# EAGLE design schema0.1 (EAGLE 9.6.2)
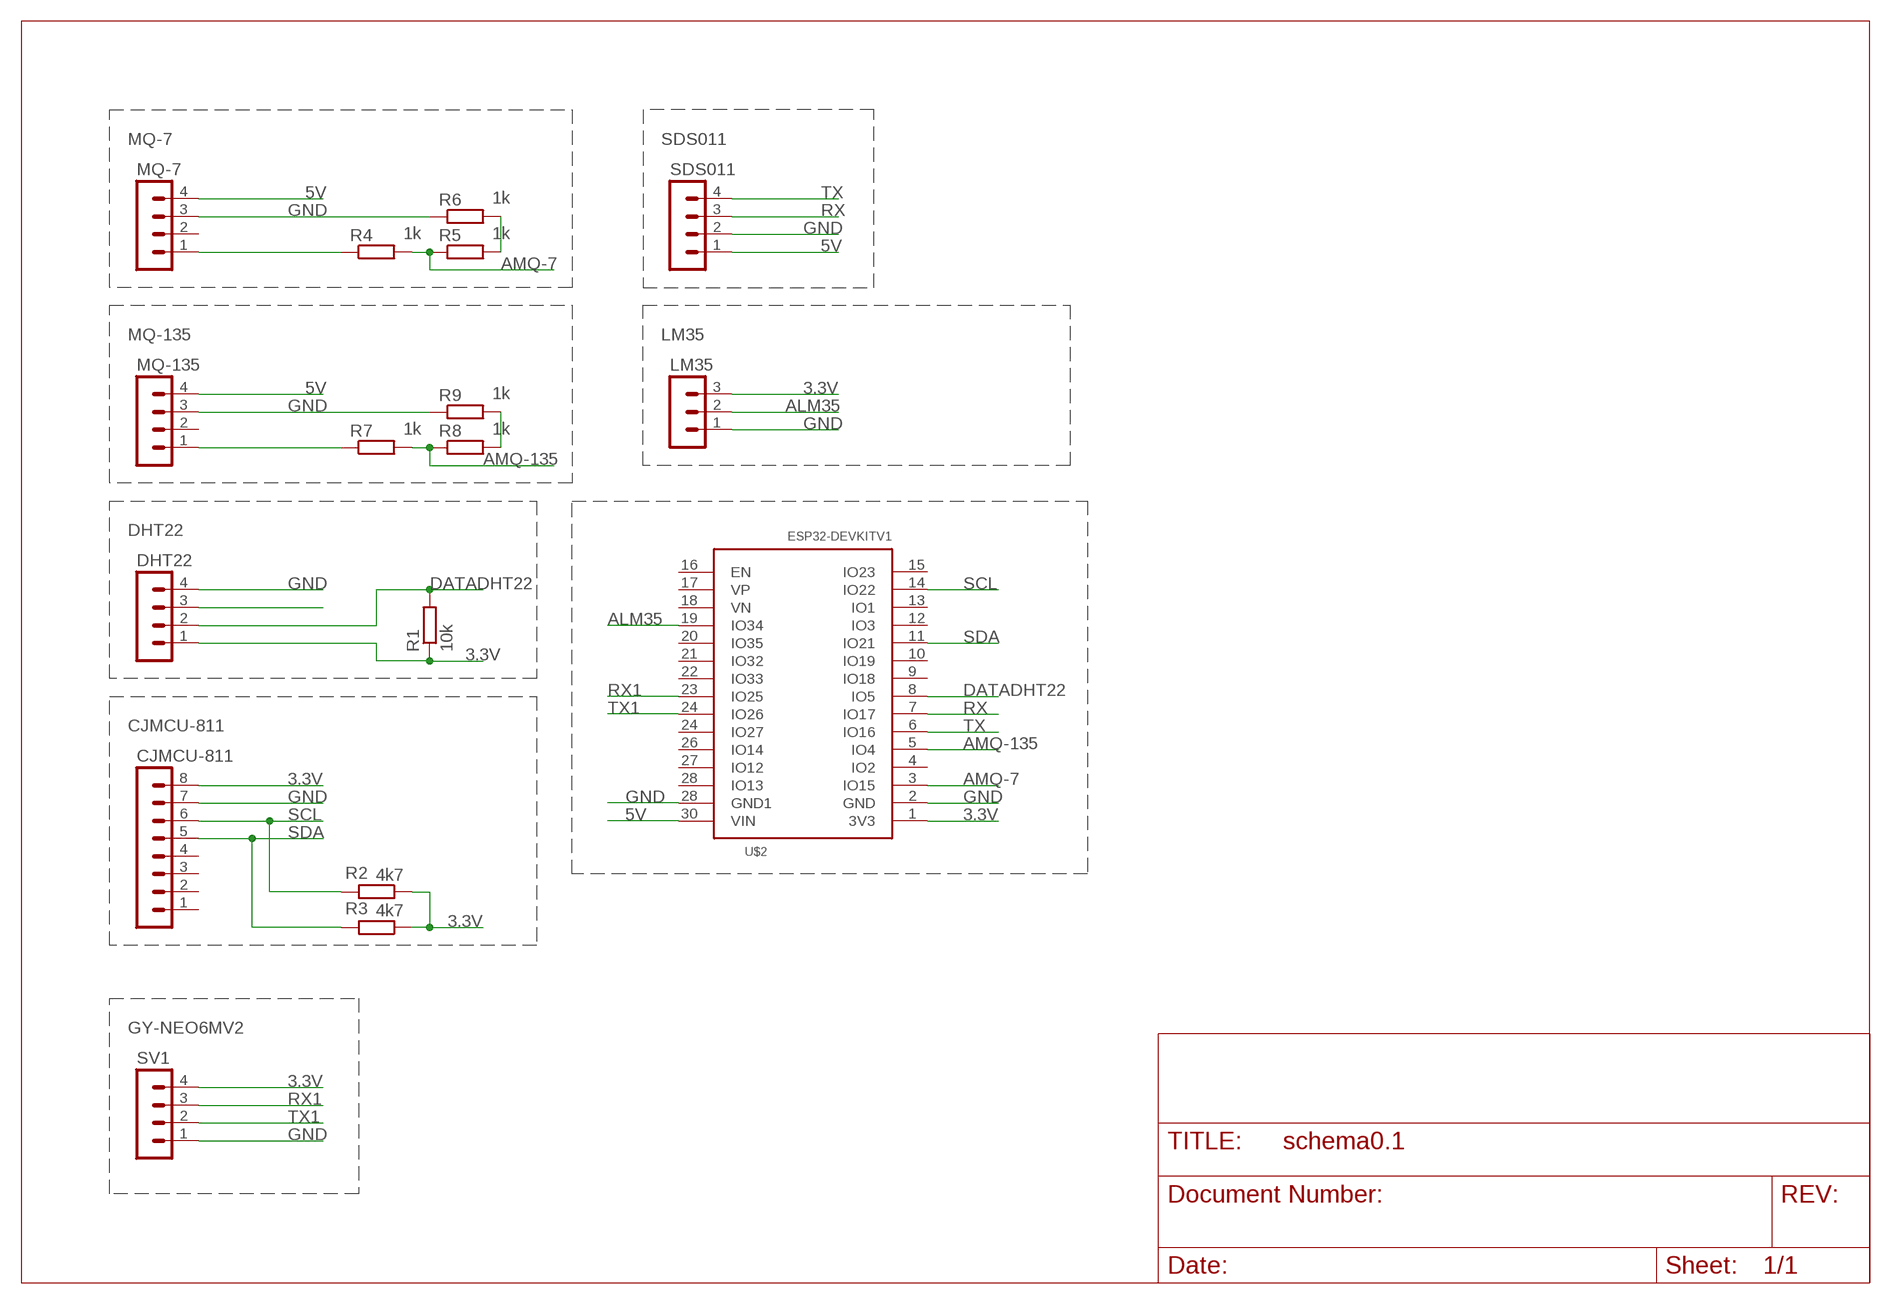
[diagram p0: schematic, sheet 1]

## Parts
CJMCU-811  MA08-1  [MA08-1]
DHT22  MA04-1  [MA04-1]
LM35  MA03-1  [MA03-1]
MQ-7  MA04-1  [MA04-1]
MQ-135  MA04-1  [MA04-1]
R1  10k  R-EU_0207/10  [0207/10]
R2  4k7  R-EU_0207/10  [0207/10]
R3  4k7  R-EU_0207/10  [0207/10]
R4  1k  R-EU_0207/10  [0207/10]
R5  1k  R-EU_0207/10  [0207/10]
R6  1k  R-EU_0207/10  [0207/10]
R7  1k  R-EU_0207/10  [0207/10]
R8  1k  R-EU_0207/10  [0207/10]
R9  1k  R-EU_0207/10  [0207/10]
SDS011  MA04-1  [MA04-1]
SV1  MA04-1  [MA04-1]
U$2  ESP32DEVKITV1  [ESP32-DEVKITV1]

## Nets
0: MQ-7.1 R4.1
1: MQ-135.1 R7.1
3.3V: CJMCU-811.8 DHT22.1 LM35.3 R1.1 R2.1 R3.1 SV1.4 U$2.1(3V3)
5V: MQ-7.4 MQ-135.4 SDS011.1 U$2.30(VIN)
ALM35: LM35.2 U$2.19(IO34)
AMQ-7: R4.2 R5.1 U$2.3(IO15)
AMQ-135: R7.2 R8.1 U$2.5(IO4)
DATADHT22: DHT22.2 R1.2 U$2.8(IO5)
GND: CJMCU-811.7 DHT22.4 LM35.1 MQ-7.3 MQ-135.3 R6.1 R9.1 SDS011.2 SV1.1 U$2.2(GND) U$2.28(GND1)
N$1: R8.2 R9.2
N$2: R5.2 R6.2
N$14: DHT22.3
RX: SDS011.3 U$2.7(IO17)
RX1: SV1.3 U$2.23(IO25)
SCL: CJMCU-811.6 R2.2 U$2.14(IO22)
SDA: CJMCU-811.5 R3.2 U$2.11(IO21)
TX: SDS011.4 U$2.6(IO16)
TX1: SV1.2 U$2.24(IO26)
Unconnected: CJMCU-811.1 CJMCU-811.2 CJMCU-811.3 CJMCU-811.4 MQ-7.2 MQ-135.2 U$2.4(IO2) U$2.9(IO18) U$2.10(IO19) U$2.12(IO3) U$2.13(IO1) U$2.15(IO23) U$2.16(EN) U$2.17(VP) U$2.18(VN) U$2.20(IO35) U$2.21(IO32) U$2.22(IO33) U$2.24(IO27) U$2.26(IO14) U$2.27(IO12) U$2.28(IO13)

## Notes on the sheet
- MQ-7 | SDS011
- MQ-135 | LM35
- DHT22
- CJMCU-811
- GY-NEO6MV2

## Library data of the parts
CJMCU-811 = con-lstb:MA08-1: PIN HEADER; OC_FARNELL: unknown; OC_NEWARK: unknown
DHT22 MQ-7 MQ-135 SDS011 SV1 = con-lstb:MA04-1: PIN HEADER; OC_FARNELL: unknown; OC_NEWARK: unknown
LM35 = con-lstb:MA03-1: PIN HEADER; OC_FARNELL: unknown; OC_NEWARK: unknown
R1-R9 = rcl:R-EU_: RESISTOR, European symbol; SPICEPREFIX: R
U$2 = ESP32-DEVKITV1:ESP32DEVKITV1

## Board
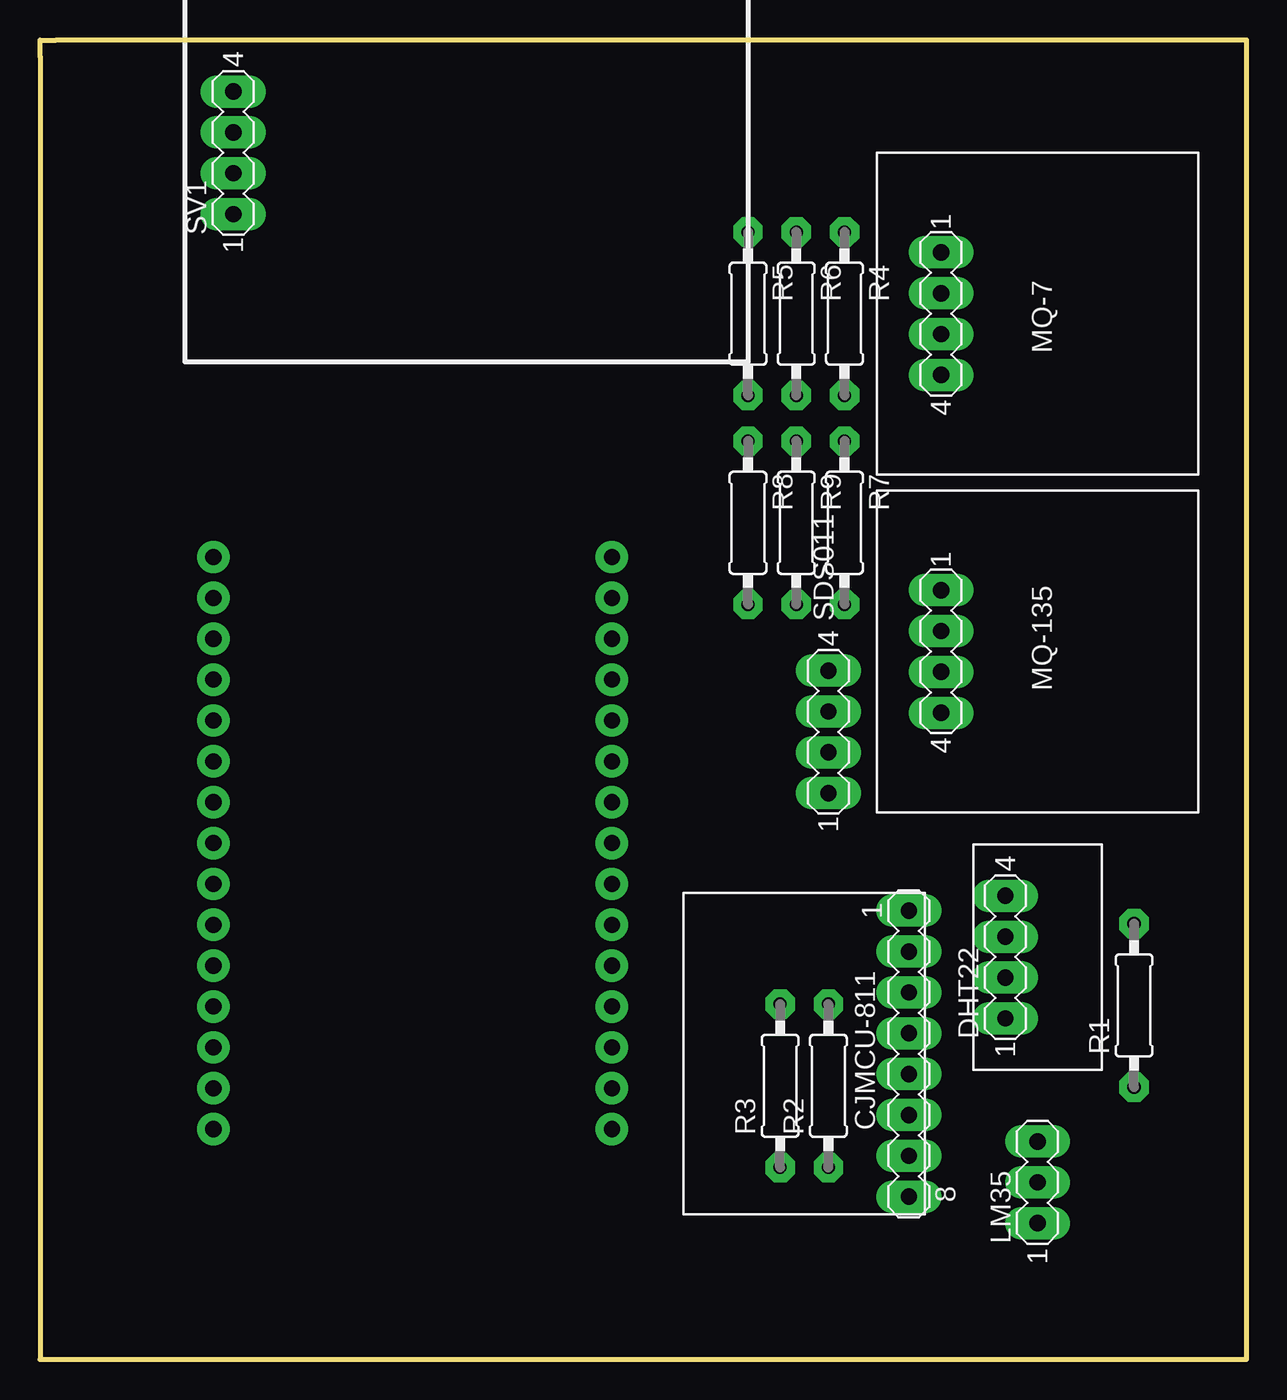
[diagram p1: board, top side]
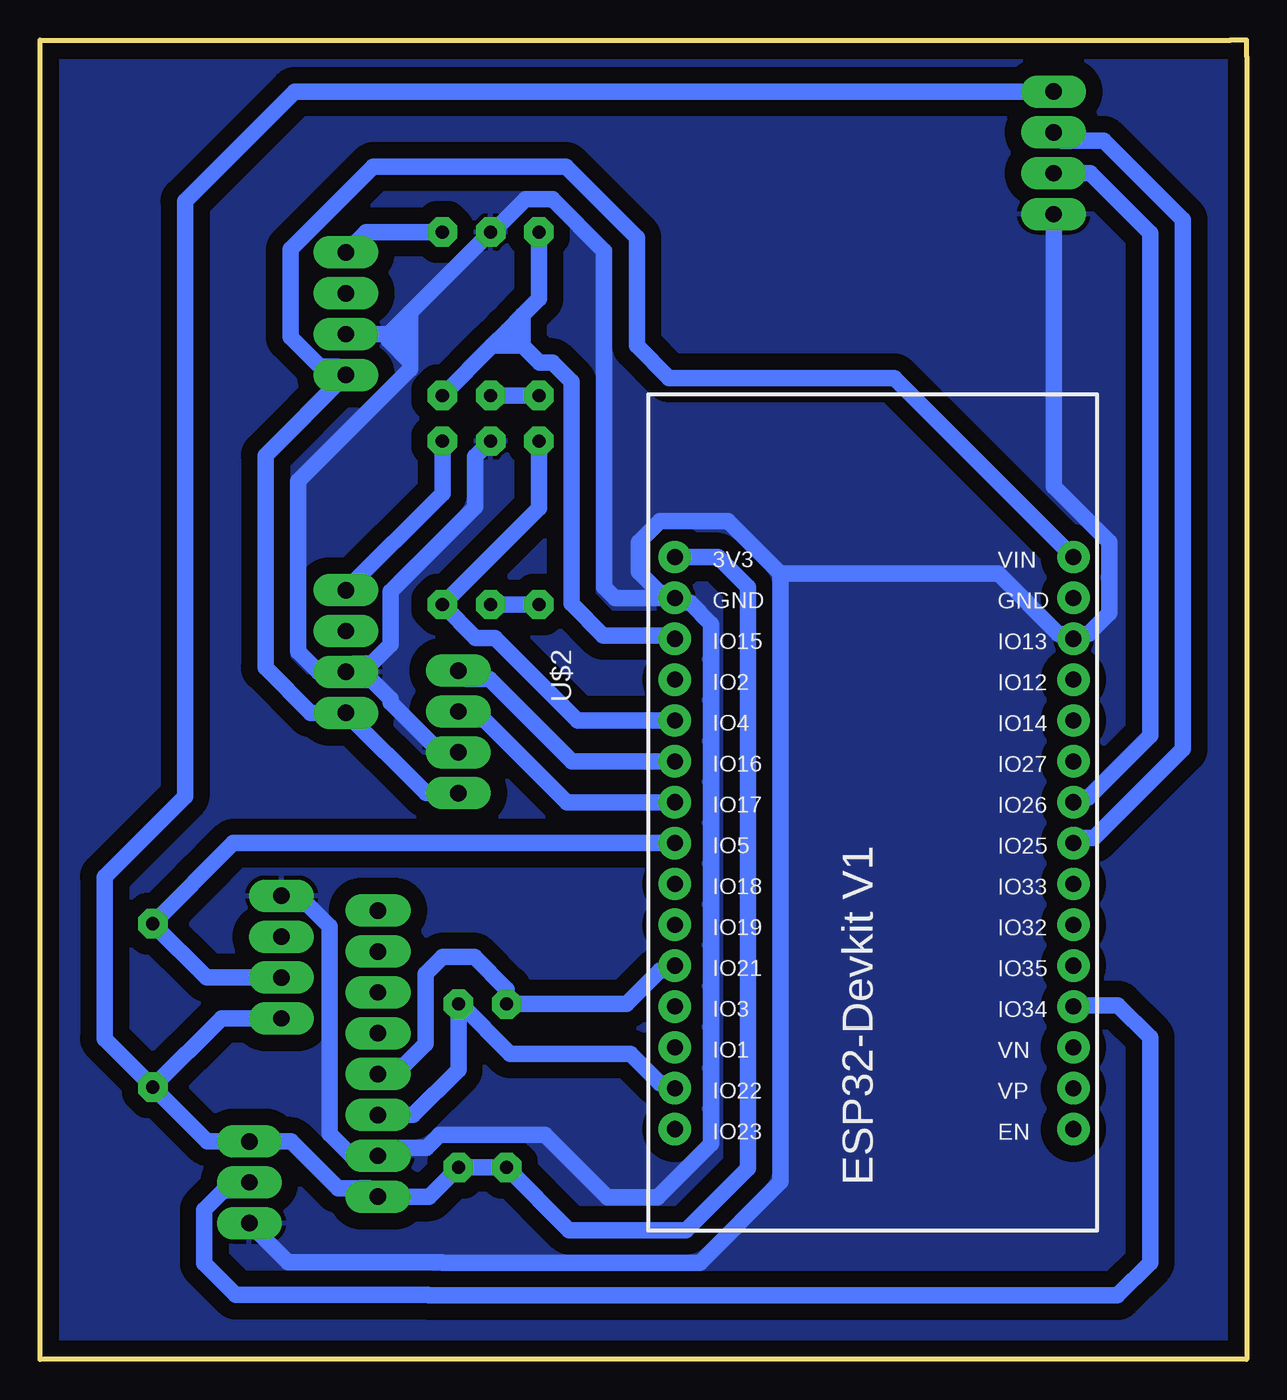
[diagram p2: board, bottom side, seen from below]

Size 75 x 82 mm. Coordinates in mm from the lower left corner, seen from the top.
Outline: 0,0 75,0 75,82 1,82 0,82 0,81 0,0
Copper layers (1*16): Top 0.035mm / dielectric 1.5mm / Bottom 0.035mm
Design rules "FreesMachien": minimum track width 40mil, minimum drill 0.4mm, track to track 40mil, track to pad 30mil, pad to pad 6mil, via to via 6mil, smd to smd 6mil, copper to edge 40mil, drill to drill 6mil, minimum pad ring 20mil, minimum via ring 20mil, stop-mask expansion 4mil, vias tented up to drill 0mil, thermal gap 10mil

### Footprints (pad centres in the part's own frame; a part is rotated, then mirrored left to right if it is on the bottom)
MA08-1 = drill 1.016 long: 1 -8.89,0; 2 -6.35,0; 3 -3.81,0; 4 -1.27,0; 5 1.27,0; 6 3.81,0; 7 6.35,0; 8 8.89,0
MA04-1 = drill 1.016 long: 1 -3.81,0; 2 -1.27,0; 3 1.27,0; 4 3.81,0
MA03-1 = drill 1.016 long: 1 -2.54,0; 2 0,0; 3 2.54,0
0207/10 = drill 0.813 octagon: 1 -5.08,0; 2 5.08,0
ESP32-DEVKITV1 = drill 1 pad 1.93: 1 -22.87,-13.54; 2 -20.33,-13.54; 3 -17.79,-13.54; 4 -15.25,-13.54; 5 -12.71,-13.54; 6 -10.17,-13.54; 7 -7.63,-13.54; 8 -5.09,-13.54; 9 -2.55,-13.54; 10 -0.01,-13.54; 11 2.53,-13.54; 12 5.07,-13.54; 13 7.61,-13.54; 14 10.15,-13.54; 15 12.69,-13.54; 16 12.69,11.23; 17 10.15,11.23; 18 7.61,11.23; 19 5.07,11.23; 20 2.53,11.23; 21 -0.01,11.23; 22 -2.55,11.23; 23 -5.09,11.23; 24 -7.63,11.23; 25 -10.17,11.23; 26 -12.71,11.23; 27 -15.25,11.23; 28 -17.79,11.23; 29 -20.33,11.23; 30 -22.87,11.23

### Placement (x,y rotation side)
CJMCU-811  54,19 270 top
DHT22  60,25 90 top
LM35  62,11 90 top
MQ-7  56,65 270 top
MQ-135  56,44 270 top
R1  68,22 90 top
R2  49,17 90 top
R3  46,17 90 top
R4  50,65 270 top
R5  44,65 270 top
R6  47,65 270 top
R7  50,52 270 top
R8  44,52 270 top
R9  47,52 270 top
SDS011  49,39 90 top
SV1  12,75 90 top
U$2  22,27 270 bottom

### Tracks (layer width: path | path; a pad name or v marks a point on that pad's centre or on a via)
0
  Bottom 1.016: R4.1 54.73,70.08 MQ-7.1
1
  Bottom 1.016: MQ-135.1 50,53.81 R7.1
3.3V
  Bottom 1.016: U$2.1 32.87,49.87 31,48 31,11.87 34.84,8.03 42.11,8.03 R3.1 R2.1 50.81,10.11 CJMCU-811.8 54.51,10.62 56.49,10.62 59.41,13.54 LM35.3 64.62,13.54 R1.1 | R1.1 63.73,21.19 DHT22.1 59.81,21 | R1.1 71,19.92 71,30 66,35 66,72 59.19,78.81 SV1.4
5V
  Bottom 1.016: SDS011.1 51,35.19 MQ-135.4 58.19,40.19 61,43 61,56.19 MQ-7.4 56.51,61.7 57.6,61.7 59.45,63.54 59.45,69 54.3,74.14 42.32,74.14 37.9,69.73 37.9,63 35.9,61 21.9,61 U$2.30
ALM35
  Bottom 1.016: U$2.19 10.84,22 8,22 6,20 6,6 8.03,3.97 50.84,3.97 50.87,4 62.84,4 64.79,5.95 64.79,9.3 63.6,10.49 62.51,10.49 LM35.2
AMQ-7
  Bottom 1.016: R4.2 46.92,63 | 46.92,63 45.96,63.96 | 45.96,63.96 45,64.92 | 45,64.92 44,65.92 R5.1 | 45,63 43.95,61.95 43.16,61.95 41.97,60.76 41.97,46.97 40,45 35.75,45 U$2.3 | 45,63 45,64.92 | 45,63 46.92,63 | 45.96,63.96 45,63
AMQ-135
  Bottom 1.016: R8.1 44,52.92 R7.2 47.92,44.84 46.73,44.84 41.6,39.71 U$2.5
DATADHT22
  Bottom 1.016: DHT22.2 64.65,23.73 R1.2 62.99,32.09 U$2.8
GND
  Bottom 1.016: MQ-7.3 53.35,63.73 | 52.04,65.04 R6.1 46.87,70.08 44.84,72.11 43.16,72.11 39.94,68.89 39.94,48 39.27,47.33 U$2.2 | 52.04,65.04 53.35,63.73 | MQ-135.3 55.49,42.22 54.4,42.22 53.21,41.03 53.21,40.84 50.1,37.73 SDS011.2 | MQ-135.3 57.7,42.73 58.97,44 58.97,54.59 52,61.55 52,62 | 52.04,65.04 52,65 52,64 | 52,62 52,64 | 53.35,63.73 52.27,63.73 52,64 | 53.35,63.73 53.35,63.35 52,62 | R9.1 47.97,56.11 47.97,52.97 53.21,47.73 53.21,44.43 54.4,43.24 55.49,43.24 MQ-135.3 | U$2.2 35.84,47.63 36.47,47.63 37.77,48.94 37.77,50.8 36.47,52.1 32.23,52.1 28.97,48.84 | 28.97,48.84 28.97,11.03 34,6 50,6 50.03,6.03 59.57,6.03 LM35.1 | 28.97,48.84 15.44,48.84 11.7,45.09 11.07,45.09 U$2.28 10.46,45.09 9.84,45.09 8.54,46.4 8.54,50.8 12,54.26 SV1.1 | DHT22.4 59.49,28.3 58.4,28.3 57,26.91 57,14 55.65,12.65 CJMCU-811.7 53.49,13.16 50.97,13.16 50.17,13.95 43.62,13.95 39.74,10.07 36.61,10.07 33.3,13.38 33.3,45.72 34.62,47.03 35.24,47.03 U$2.2
  pour Bottom: 66,79 66,3 5,3 5,79
KOPER
  pour Bottom: 0,82 75,82 75,0 0,0
N$1
  Bottom 1.016: R8.2 R9.2
N$2
  Bottom 1.016: R5.2 R6.2
RX
  Bottom 1.016: SDS011.3 48.49,39.76 47.4,39.76 42.26,34.63 U$2.7
RX1
  Bottom 1.016: SV1.3 11.49,75.76 8.89,75.76 3.97,70.84 3.97,37.94 9.51,32.4 10.46,32.4 U$2.23
SCL
  Bottom 1.016: CJMCU-811.6 51.81,15.19 49,18 R2.2 48.87,22.08 45.79,19 38.31,19 36.47,17.16 35.84,17.16 U$2.14
SDA
  Bottom 1.016: CJMCU-811.5 53.49,18.24 52.4,18.24 51.03,19.6 51.03,23.97 50,25 48,25 46,23 R3.2 38.55,22.08 36.47,24.16 35.84,24.16 U$2.11
TX
  Bottom 1.016: SDS011.4 48.49,42.3 47.06,42.3 41.93,37.17 U$2.6
TX1
  Bottom 1.016: U$2.24 10.46,34.94 9.84,34.94 6,38.78 6,70 9.73,73.73 SV1.2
